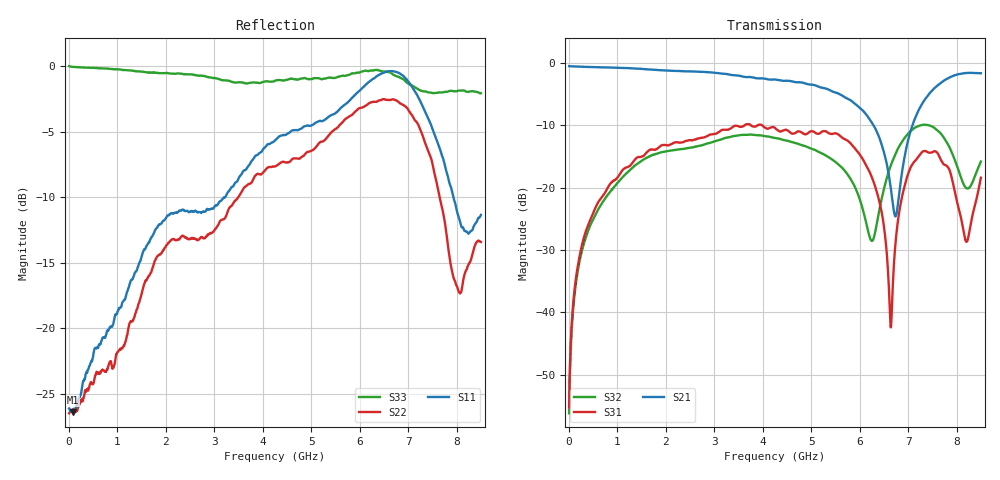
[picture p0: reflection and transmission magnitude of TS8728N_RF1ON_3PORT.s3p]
!Created with skrf (http://scikit-rf.org).
# GHz S RI R 50.0
!freq ReS11 ImS11 ReS12 ImS12 ReS13 ImS13
! ReS21 ImS21 ReS22 ImS22 ReS23 ImS23
! ReS31 ImS31 ReS32 ImS32 ReS33 ImS33
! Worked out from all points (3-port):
!   1601 points, 10 MHz to 8.5 GHz, reference 50 ohm
!   strongest paths, dB at 10 MHz, 2.132 GHz, 4.255 GHz, 6.378 GHz, 8.5 GHz:
!     S21: -0.5, -1.2, -2.6, -11.4, -1.6
!     S31: -55.2, -12.9, -10.4, -21.3, -18.4
!     S32: -56.2, -14.0, -12.0, -24.8, -15.8
!   lowest |S11| = -26.4 dB at 94.9 MHz (marker M1), VSWR 1.10, Z = 54.6 - j2.04 ohm
!   |S11| at or under -10 dB: start of sweep to 3.228 GHz; 7.932 GHz to end of sweep
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0.01  0.0495 -0.00161  0.9456 -0.00641  0.000667 0.00157
      0.9456 -0.00659  0.0475 -0.00103  0.00063 0.00143
      0.000687 0.00159  0.000586 0.00144  0.9977 -0.0107
0.0949  0.0441 -0.0187  0.9399 -0.0415  0.00164 0.0118
        0.9402 -0.0414  0.0458 -0.0179  0.00155 0.0107
        0.0016 0.0118  0.00158 0.0107  0.9879 -0.0798
2.00515  -0.1195 -0.2342  0.6136 -0.6224  0.2055 0.0789
         0.6132 -0.6231  -0.1693 -0.1166  0.1938 0.0305
         0.2058 0.0788  0.1935 0.0306  0.0783 -0.9357
4.255  -0.4849 -0.188  -0.0657 -0.7364  0.1977 -0.2287
       -0.0669 -0.7366  -0.3236 0.2584  0.0914 -0.2343
       0.1971 -0.2292  0.0918 -0.234  -0.8493 -0.2259
6.0379  -0.7539 0.3174  -0.3772 -0.2003  -0.0958 -0.1484
        -0.3771 -0.2003  0.2248 0.655  -0.0415 -0.0605
        -0.0956 -0.1483  -0.0416 -0.0605  -0.4806 0.8198
6.626894  -0.6937 0.656  -0.1031 -0.0378  -0.00338 -0.00881
          -0.103 -0.0378  0.6368 0.3793  0.116 -0.0869
          -0.00339 -0.00881  0.1159 -0.0872  -0.046 0.9432
7.109763  -0.2304 0.7847  0.1694 -0.288  0.1239 -0.0991
          0.1697 -0.2885  0.6268 -0.0989  0.0798 -0.287
          0.1241 -0.0992  0.0801 -0.2868  0.4337 0.715
7.884475  0.1223 0.322  -0.2269 -0.7441  -0.0851 -0.0941
          -0.2274 -0.7432  -0.0231 -0.1709  -0.1514 -0.1285
          -0.0851 -0.0938  -0.1517 -0.1285  0.7887 -0.1547
8.20285  -0.0251 0.2325  -0.4849 -0.6774  -0.0193 0.0314
         -0.4856 -0.6771  -0.1638 0.0355  -0.0474 -0.087
         -0.0193 0.0314  -0.0472 -0.0874  0.5308 -0.5955
8.5  -0.1552 0.2217  -0.6347 -0.534  0.111 0.047
     -0.635 -0.5338  -0.1115 0.1819  0.0124 -0.1622
     0.111 0.0471  0.0127 -0.162  0.0709 -0.7834
